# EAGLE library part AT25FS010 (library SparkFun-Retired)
1-Mbit SPI flash memory Retired: IC-09350
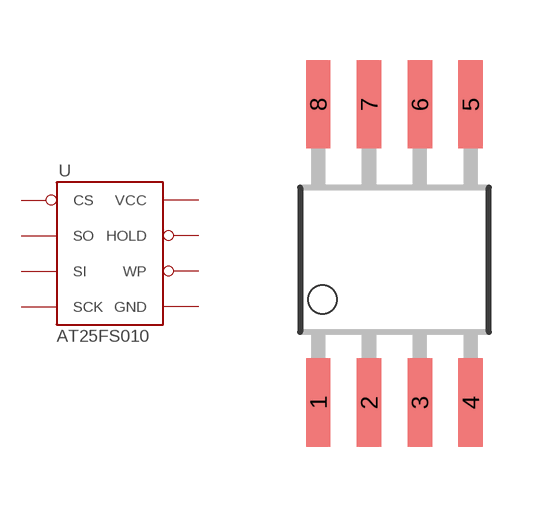
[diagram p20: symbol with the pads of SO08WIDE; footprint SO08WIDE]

Designator prefix -

## AT25FS010  [SO08WIDE]
1  CS
2  SO
3  WP
4  GND
5  SI
6  SCK
7  HOLD
8  VCC

## Footprint SO08WIDE (pad centres in mm)
smd 0.61 x 2.21: 1 -1.905,-3.569; 2 -0.635,-3.569; 3 0.635,-3.569; 4 1.905,-3.569; 5 1.905,3.886; 6 0.635,3.886; 7 -0.635,3.886; 8 -1.905,3.886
